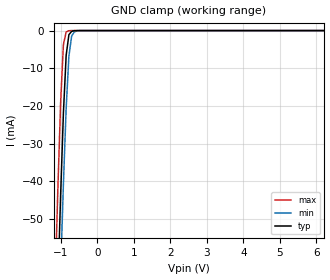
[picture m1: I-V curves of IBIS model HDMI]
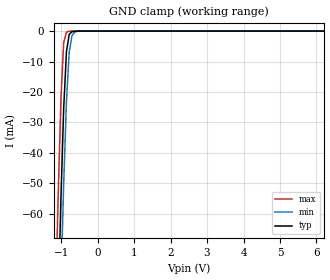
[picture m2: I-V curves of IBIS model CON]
| Texas Instruments Incorporated
| 13 Channel ESD Protection Solution with Current-Limit Load Switch for
| HDMI Port
| Marketing part#   Voltage Range   Package-type   #pins/pkg drawing
| TPD13S523PWR   5V   TSSOP   16-pin PWR
[IBIS Ver]   4.0
[File name]   tpd13s523.ibs
[File Rev]   1.0
[Date]   07/20/2011
[Source]   TIspiceD simulations
   Texas Instruments Incorporated.
   Analog eLab Design Center, HPA
   12500 TI Blvd
   Dallas, TX -75243
   For Support e-mail: elab_scm_ibis@list.ti.com
[Notes]   Revision History:
   Rev 1.0: 07/20/2011
   - C_comp although listed in numerical order of value are
   obtained from varying PVT conditions.
   For PVT conditions for each specific value, refer to the
   buffer description under respective [Model].
   IBIS model user is responsible for using appropriate
   C_comp to simulate for Signal Integrity.
   - IBIS model not matched to TISPICED simulations
[Disclaimer] This model is designed as an aid for customers of Texas Instruments.
 TI and its licensors and suppliers make no warranties, either expressed
 or implied, with respect to this  model, including the warranties of
 merchantability or fitness for a particular purpose.
 The model is provided solely on an "as is" basis. The entire risk as to
 its quality and performance is with the customer.
[Copyright] (C)Copyright 2011 Texas Instruments Incorporated.
   All rights reserved.
|   Component TPD13S523PWR
[Component]   TPD13S523PWR
[Manufacturer]  Texas Instruments Incorporated
[Package]   |(PWR) 16-pin TSSOP
|   typ   min   max
R_pkg   0.726922   0.68468   0.78309
L_pkg   3.326317nH   2.97366nH   3.68543nH
C_pkg   0.494424pF   0.45875pF   0.53395pF
[Pin]   signal_name   model_name   R_pin   L_pin   C_pin
1   CEC   CON   0.68468   3.67539nH   0.53264pF
2   UTILITY   CON   0.78309   3.47819nH   0.51884pF
3   DDC_DAT   CON   0.74487   3.15196nH   0.45901pF
4   DDC_CLK   CON   0.68736   2.97422nH   0.46201pF
5   5V_SUPPLY   POWER   0.37906   2.56622nH   0.50947pF
6   5V_OUT   POWER   0.40039   2.68455nH   0.50581pF
7   HPD_DET   CON   0.75169   3.39049nH   0.51239pF
8   GND   GND   0.7153   3.77496nH   0.53534pF
9   D3N   HDMI   0.68572   3.68543nH   0.53395pF
10   D3P   HDMI   0.78083   3.4768nH   0.51935pF
11   D2N   HDMI   0.7436   3.15186nH   0.4588pF
12   D2P   HDMI   0.68688   2.97409nH   0.45984pF
13   D1N   HDMI   0.68719   2.97366nH   0.45981pF
14   D1P   HDMI   0.74439   3.15059nH   0.45875pF
15   D0N   HDMI   0.78229   3.47561nH   0.51894pF
16   D0P   HDMI   0.6874   3.68383nH   0.53318pF
[Diff_pin]   inv_pin   vdiff   tdelay_typ   tdelay_min   tdelay_max
|Vidff not present in datasheet
|Vdiff is not applicable as these are just ESD diff pins
|hence NA for vdiff
16   15   NA   0 0 0
14   13   NA   0 0 0
12   11   NA   0 0 0
10   9   NA   0 0 0
| Models and submodels in the file (2): HDMI (Input), CON (Input)
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[Model]   HDMI
Model_type   Input
|  Diode forward voltage
Vinl = 0.6V
Vinh = 0.95V
|   typ   min   max
|   (nom)   (slow)   (fast)
C_comp   0.77513pF   0.77251pF   0.77785pF
[Voltage Range]   5.000V   5.00V   5.00V
|Junction temperature
[Temperature Range]   40.0   100.0   -40.0
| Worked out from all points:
|   GND clamp passes 1 mA (typ) near -0.77 V on its own axis
|ambient temperature   25   85   -40|
[GND Clamp]
|   Voltage   I(typ)   I(min)   I(max)
-5V       -1.553A    -1.571A    -1.532A
-1.156V   -93.56mA   -114.8mA   -67mA
-1.08V    -67.86mA   -88.95mA   -41.67mA
-1.005V   -43.54mA   -64.04mA   -18.96mA
-929.6mV  -21.95mA   -40.77mA   -3.749mA
-854.3mV  -6.576mA   -20.63mA   -366.4uA
-778.9mV  -1.084mA   -6.767mA   -35.31uA
-703.5mV  -203.1uA   -1.444mA   -1.065uA
-628.1mV  -25.36uA   -333.1uA   -25.63nA
-477.4mV  -110.8nA   -7.927uA   -17.51pA
10V       0A         0A         0A
[POWER Clamp]
|   Voltage   I(typ)   I(min)   I(max)
-5V       0A         0A         0A
0V        0A         0A         0A
10V       0A         0A         0A
[Model]   CON
Model_type   Input
|  Diode forward voltage
Vinl = 0.6V
Vinh = 0.95V
|   typ   min   max
|   (nom)   (slow)   (fast)
C_comp   0.70449pF   0.70218pF   0.70677pF
[Voltage Range]   5.000V   5.00V   5.00V
|Junction temperature
[Temperature Range]   40.0   100.0   -40.0
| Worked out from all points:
|   GND clamp passes 1 mA (typ) near -0.77 V on its own axis
|ambient temperature   25   85   -40|
[GND Clamp]
|   Voltage   I(typ)   I(min)   I(max)
-5V       -2.265A    -2.289A    -2.236A
-1.156V   -126.8mA   -156.2mA   -90.33mA
-1.08V    -89.68mA   -118.7mA   -53.89mA
-1.005V   -55.03mA   -82.98mA   -22.3mA
-929.6mV  -25.48mA   -50.25mA   -3.811mA
-854.3mV  -6.809mA   -23.36mA   -378.2uA
-778.9mV  -1.101mA   -6.987mA   -37.2uA
-703.5mV  -212.2uA   -1.467mA   -1.125uA
-628.1mV  -26.71uA   -346.4uA   -27.14nA
-477.4mV  -117.4nA   -8.36uA    -19.54pA
10V       0A         0A         0A
[POWER Clamp]
|   Voltage   I(typ)   I(min)   I(max)
-5V       0A         0A         0A
0V        0A         0A         0A
10V       0A         0A         0A
